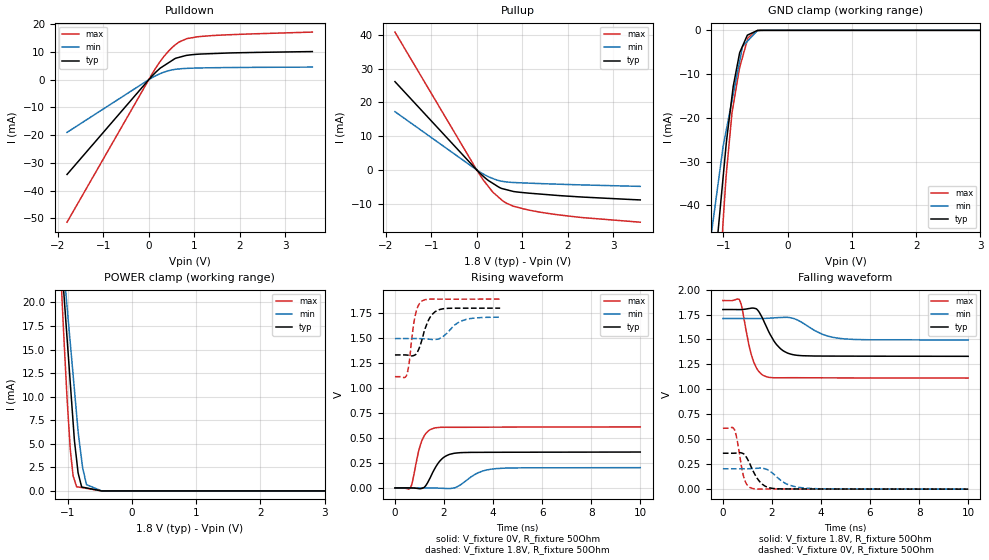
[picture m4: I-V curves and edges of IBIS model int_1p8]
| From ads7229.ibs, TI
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|   int_1p8 Model
[Model]   int_1p8
Model_type   I/O
Polarity   Non-Inverting
Enable   Active-Low
Vinl = 0.63
Vinh = 1.17
Vmeas = 0.9
Vref = 0.9
Cref = 30pF
Rref = 50
|   typ   min   max
|   (nom PVT)   (Fast PVT)   (slow PVT)
|C_comp from frequency sweep method(F=50MHz)
C_comp   5.726e-12   4.640e-12   6.678e-12
|OFF state: BUFFER IN HIGH IMPEDANCE
|C_comp   5.726e-12   4.640e-12   6.678e-12
|ON state : BUFFER OUTPUT TURNED HIGH
|C_comp   5.469e-12   4.378e-12   6.396e-12
|C_comp from LC tank measurement(L=1nH)
|ON state : BUFFER OUTPUT TURNED HIGH
|Resonant Frequency(Hz)   2.500e+09   2.690e+09   2.330e+09
|C_comp   4.057e-12   3.504e-12   4.670e-12
|OFF state: BUFFER IN HIGH IMPEDANCE
|Resonant Frequency   2.520e+09   2.760e+09   2.340e+09
|C_comp   3.993e-12   3.329e-12   4.631e-12
| Where nom  PVT is Nominal Process,  1.8V,  28C
|   Fast PVT is Strong Process,   1.89V,  -40C
|   Slow PVT is Weak Process,   1.71V,  88C
[Model Spec]
|Subparameter   typ   min   max
Vinh   1.17   1.1115   1.2285
Vinl   0.63   0.5985   0.6615
[Voltage Range]   1.8   1.71   1.89
|Ambient Temperature   25   85   -40
|Junction Temperature
[Temperature Range]   28   88   -40
[Pullup Reference]   1.8   1.71   1.89
[Pulldown Reference]   0   0   0
[Power Clamp Reference]   1.8   1.71   1.89
[GND Clamp Reference]   0   0   0
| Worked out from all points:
|   slope of the pulldown table from 0 to 0.27 V, typ, clamps not added: 62 ohm
|   slope of the pullup table from 0 to 0.27 V, typ, clamps not added: 83 ohm
|   GND clamp passes 1 mA (typ) near -0.61 V on its own axis
|   POWER clamp passes 1 mA (typ) near -0.80 V on its own axis
|   falling waveform, V_fixture 1.8V, R_fixture 50Ohm: 20-80 % time 652ps typ, 977ps min, 426ps max; typ from 1.8 V to 1.33 V
|   rising waveform, V_fixture 0V, R_fixture 50Ohm: 20-80 % time 528ps typ, 773ps min, 364ps max; typ from 0 V to 0.359 V
|   rising waveform, V_fixture 1.8V, R_fixture 50Ohm: 20-80 % time 401ps typ, 606ps min, 247ps max; typ from 1.33 V to 1.8 V
|   falling waveform, V_fixture 0V, R_fixture 50Ohm: 20-80 % time 482ps typ, 699ps min, 267ps max; typ from 0.361 V to 0.001 V
[Pulldown]
|   Voltage   I(typ)   I(min)   I(max)
-1.8V     -34.19mA   -19.02mA   -51.42mA
107.7mV   1.924mA    1.041mA    3.045mA
252mV     4.165mA    2.161mA    6.604mA
332.6mV   5.019mA    2.694mA    8.371mA
449.8mV   6.26mA     3.286mA    10.58mA
574.6mV   7.581mA    3.708mA    12.48mA
665.3mV   8.048mA    3.86mA     13.56mA
833.5mV   8.756mA    4.065mA    14.78mA
1.087V    9.182mA    4.201mA    15.5mA
1.784V    9.633mA    4.368mA    16.21mA
3.6V      10.13mA    4.532mA    17.16mA
[GND Clamp]
|   Voltage   I(typ)   I(min)   I(max)
-1.8V     -186.4mA   -124.5mA   -273.1mA
-1.228V   -71.67mA   -50.84mA   -103.3mA
-1.105V   -49.28mA   -37.39mA   -69.41mA
-1.07V    -43.69mA   -33.52mA   -59.66mA
-1.005V   -33.55mA   -26.51mA   -43.65mA
-958.2mV  -26.1mA    -22.92mA   -33.24mA
-867.5mV  -15.12mA   -16.08mA   -18.88mA
-748.8mV  -5.178mA   -7.133mA   -8.512mA
-702.8mV  -3.601mA   -3.665mA   -6.109mA
-628.2mV  -1.099mA   -2.502mA   -2.221mA
-456.6mV  -26.53uA   -27.48uA   -23.27uA
3.6V      0A         0A         0A
[Pullup]
|   Voltage   I(typ)   I(min)   I(max)
-1.8V     26.13mA    17.26mA    40.8mA
0V        0A         0A         0A
139.9mV   -1.824mA   -1.172mA   -2.9mA
332.6mV   -3.783mA   -2.419mA   -6.214mA
495mV     -5.16mA    -3.174mA   -8.234mA
574.6mV   -5.573mA   -3.408mA   -9.177mA
801.4mV   -6.351mA   -3.712mA   -10.71mA
1.164V    -6.89mA    -3.919mA   -11.92mA
1.542V    -7.297mA   -4.105mA   -12.81mA
2.362V    -8.051mA   -4.448mA   -14.14mA
3.6V      -8.875mA   -4.87mA    -15.46mA
[POWER Clamp]
|   Voltage   I(typ)   I(min)   I(max)
-1.8V     100.6mA    87.32mA    118.7mA
-1.086V   24.01mA    25.53mA    20.2mA
-1.058V   20.94mA    23.36mA    16.3mA
-1.009V   16.27mA    19.58mA    9.855mA
-958.2mV  11.41mA    15.66mA    4.395mA
-914.8mV  7.282mA    12.31mA    1.606mA
-859.9mV  3.29mA     8.1mA      443.7uA
-837mV    1.908mA    6.336mA    417.5uA
-781.2mV  415uA      3.267mA    354uA
-706.2mV  314.5uA    666.7uA    268.5uA
-470.3mV  35.57nA    528.3nA    0A
3.6V      0A         0A         0A
[Ramp]
R_load = 50
|   typ   min   max
dV/dt_r   0.21549/5.27728e-10   0.121754/7.67458e-10   0.366398/3.62095e-10
dV/dt_f   0.281238/6.46159e-10   0.128964/9.72389e-10   0.466039/4.25691e-10
[Falling Waveform]
V_fixture = 1.8V
V_fixture_min = 1.71V
V_fixture_max = 1.89V
R_fixture = 50Ohm
|   Time   V(typ)   V(min)   V(max)
0s        1.8V       1.71V      1.89V
674ps     1.799V     1.71V      1.898V
776ps     1.8V       1.71V      1.82V
1.237ns   1.814V     1.71V      1.289V
1.462ns   1.78V      1.71V      1.18V
1.799ns   1.615V     1.712V     1.125V
2.339ns   1.41V      1.72V      1.116V
2.922ns   1.345V     1.707V     1.117V
4.693ns   1.333V     1.513V     1.115V
10ns      1.331V     1.495V     1.113V
[Rising Waveform]
V_fixture = 0V
V_fixture_min = 0V
V_fixture_max = 0V
R_fixture = 50Ohm
|   Time   V(typ)   V(min)   V(max)
0s        738.9pV    916.9pV    608.3pV
626ps     460.5uV    8.463uV    2.433mV
1.101ns   -4.252mV   238uV      474.5mV
1.336ns   54.93mV    376.8uV    564.2mV
1.616ns   190.3mV    -408.1uV   599.6mV
2.038ns   314mV      -4.911mV   607mV
2.655ns   352.8mV    28.58mV    606.5mV
3.387ns   356.1mV    151.3mV    607.4mV
4.117ns   356.7mV    193.4mV    608.2mV
10ns      359.2mV    202.9mV    610.7mV
[Rising Waveform]
V_fixture = 1.8V
V_fixture_min = 1.71V
V_fixture_max = 1.89V
R_fixture = 50Ohm
|   Time   V(typ)   V(min)   V(max)
0s        1.33V      1.494V     1.113V
474ps     1.329V     1.494V     1.126V
572ps     1.327V     1.494V     1.24V
796ps     1.328V     1.494V     1.689V
926ps     1.364V     1.494V     1.81V
1.094ns   1.476V     1.493V     1.868V
1.418ns   1.701V     1.487V     1.889V
1.785ns   1.781V     1.491V     1.888V
2.734ns   1.798V     1.672V     1.888V
4.289ns   1.798V     1.708V     1.889V
[Falling Waveform]
V_fixture = 0V
V_fixture_min = 0V
V_fixture_max = 0V
R_fixture = 50Ohm
|   Time   V(typ)   V(min)   V(max)
0s        360.5mV    204.5mV    611.1mV
472ps     360.7mV    204.2mV    596.4mV
871ps     348.9mV    204.3mV    105.2mV
1.005ns   300.6mV    204.9mV    37.17mV
1.22ns    187.2mV    206.9mV    6.506mV
1.605ns   50.05mV    210.1mV    1.43mV
2.19ns    4.48mV     123.4mV    2.392mV
2.631ns   2.352mV    48.84mV    2.111mV
3.391ns   2.217mV    10.21mV    1.62mV
10ns      732.2uV    979.2uV    225.9uV
